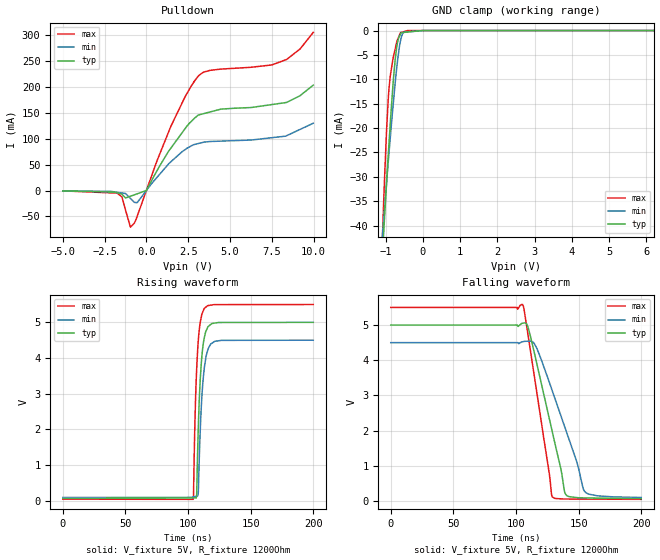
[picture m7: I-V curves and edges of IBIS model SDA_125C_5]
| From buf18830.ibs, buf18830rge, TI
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|   SDA_5 Model
[Model] SDA_125C_5
|Signals SDA(15)
Model_type   I/O_open_drain
Polarity   Non-Inverting
Enable   Active-Low
Vinl = 1.5
Vinh = 3.5
Vmeas = 2.5
Vref = 2.5
Cref = 0pF
Rref = 10000
| Rpullup to DVDD = 1k
|   typ   min   max
|   (Nom PVT)   (Slow PVT)   (Fast PVT)
|   Output Low
|C_comp   9.55169E-13   8.2429E-13   1.16434E-12
|   Output High
C_comp   1.06189E-12   9.46412E-13   1.2305E-12
| Where   Nom PVT is  Nominal Process, 5.0V, 57C
|   Fast PVT is Strong Process, 5.5V, -40C
|   Slow PVT is Weak Process, 4.5V, 125C
[Model Spec]   |5V model
Vinl   1.5   1.35   1.65
Vinh   3.5   3.15   3.85
|Vinl = 0.3 X DVDD
|Vinh = 0.7 X DVDD
[Voltage Range]   5   4.5   5.5
|Operating Temperature   27   85   -40
[Temperature Range]   67   125   -40
[Pullup Reference]   5   4.5   5.5
[Pulldown Reference]   0   0   0
[Power Clamp Reference]   5   4.5   5.5
[GND Clamp Reference]   0   0   0
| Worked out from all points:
|   slope of the pulldown table from 0 to 0.75 V, typ, clamps not added: 16.7 ohm
|   GND clamp passes 1 mA (typ) near -0.62 V on its own axis
|   falling waveform, V_fixture 5V, R_fixture 1200Ohm: 20-80 % time 19ns typ, 25.4ns min, 14.1ns max; typ from 5 V to 0.069 V
|   rising waveform, V_fixture 5V, R_fixture 1200Ohm: 20-80 % time 3.52ns typ, 3.87ns min, 3.17ns max; typ from 0.068 V to 5 V
[Pulldown]
|   Voltage   I(typ)   I(min)   I(max)
-5V       -659.3uA   -493.7uA   -664.8uA
-1.737V   -4.54mA    -3.417mA   -5.099mA
-1.46V    -7.292mA   -4.747mA   -12.59mA
-952.8mV  -11.01mA   -15.23mA   -70.84mA
-563.1mV  -6.499mA   -23.51mA   -50.92mA
404.1uV   25.46uA    16.32uA    38.17uA
1.458V    81.73mA    55.42mA    123.7mA
2.316V    119.7mA    79.08mA    181.4mA
3.148V    146.4mA    91.26mA    222.7mA
8.392V    170.5mA    106.1mA    253.6mA
9.205V    183.8mA    118.4mA    274.1mA
9.985V    203.8mA    130.2mA    306mA
[GND Clamp]
|   Voltage   I(typ)   I(min)   I(max)
-5V       -603.5mA   -445.1mA   -1.001A
-1.127V   -51.08mA   -45.8mA    -50.73mA
-1.045V   -40.22mA   -37.88mA   -33.25mA
-976.1mV  -31.18mA   -31.29mA   -20.46mA
-929.4mV  -25.42mA   -26.79mA   -13.83mA
-876.6mV  -19.06mA   -22.04mA   -9.344mA
-738.9mV  -5.548mA   -10.31mA   -3.591mA
-684.4mV  -2.565mA   -6.406mA   -1.931mA
-597.1mV  -700.3uA   -1.977mA   -414.4uA
-516.7mV  -390.3uA   -315.6uA   -237.6uA
-813.9uV  -919.2nA   0A         0A
9.985V    0A         0A         0A
[POWER Clamp]
|   SCR cell for ESD function. Effects occurr above VDD x 2
|   Voltage   I(typ)   I(min)   I(max)
-5V       0A         0A         0A
0V        0A         0A         0A
10V       0A         0A         0A
[Ramp]
R_load = 1200
|   typ   min   max
dV/dt_r   2.95936/3.51139e-009   2.64276/3.86302e-009   3.27084/3.17132e-009
dV/dt_f   2.95869/1.89763e-008   2.63957/2.54082e-008   3.27074/1.40555e-008
[Falling Waveform]
V_fixture = 5V
V_fixture_min = 4.5V
V_fixture_max = 5.5V
R_fixture = 1200Ohm
C_fixture = 0F
|   Time   V(typ)   V(min)   V(max)
0s        5V         4.5V       5.5V
101.3ns   4.982V     4.5V       5.448V
105.3ns   5.051V     4.525V     5.584V
108.9ns   5.004V     4.54V      4.876V
114.6ns   4.219V     4.476V     3.552V
129ns     1.971V     3.132V     120.1mV
139.6ns   192.9mV    2.038V     57.9mV
148.7ns   98.39mV    1.1V       56.53mV
154.9ns   89.8mV     271.4mV    55.59mV
200ns     68.84mV    100.7mV    48.77mV
[Rising Waveform]
V_fixture = 5V
V_fixture_min = 4.5V
V_fixture_max = 5.5V
R_fixture = 1200Ohm
C_fixture = 0F
|   Time   V(typ)   V(min)   V(max)
0s        67.74mV    95.39mV    48.59mV
104.1ns   83.77mV    111.5mV    44.13mV
105.5ns   83.98mV    120.9mV    2.168V
106.8ns   119mV      130.4mV    3.625V
107.5ns   1.191V     135.5mV    4.141V
108.2ns   2.089V     255.2mV    4.501V
109.8ns   3.452V     2.056V     5.02V
112.8ns   4.538V     3.655V     5.379V
121.3ns   4.98V      4.469V     5.497V
200ns     5V         4.5V       5.5V
